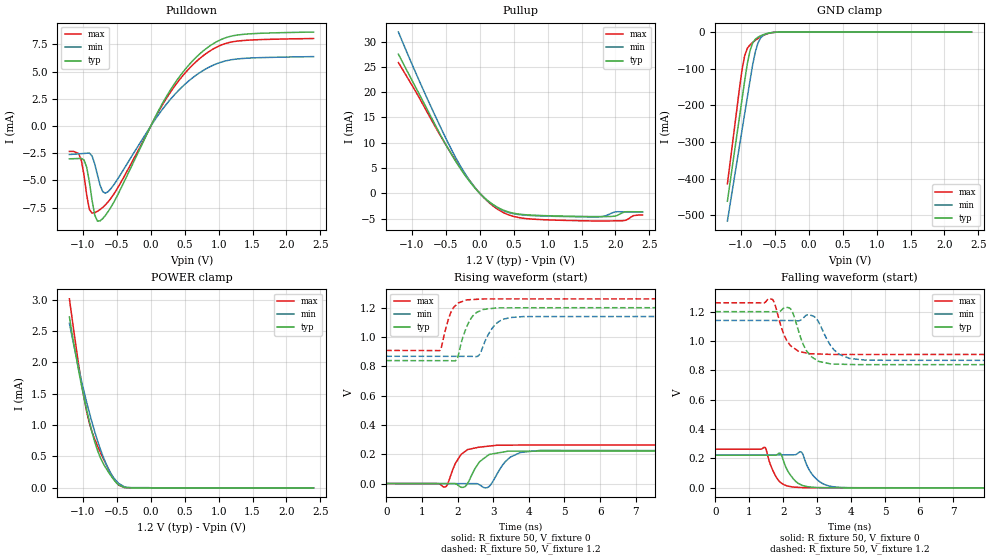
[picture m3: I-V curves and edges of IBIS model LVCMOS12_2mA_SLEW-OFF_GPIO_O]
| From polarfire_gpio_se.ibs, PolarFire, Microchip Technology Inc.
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|   Model LVCMOS12_2mA_SLEW-OFF_GPIO_O
[Model]   LVCMOS12_2mA_SLEW-OFF_GPIO_O
Model_type   Output
Polarity   Non-Inverting
Enable   Active-High
Vmeas =   0.6
Cref =   5p
Rref =   1M
|   typ   min   max
C_comp_pullup   2.605e-12   2.605e-12   2.76e-12
C_comp_pulldown  2.605e-12   2.605e-12   2.76e-12
[Temperature Range]  25C   100C   -40C
[Voltage Range]  1.2   1.14   1.26
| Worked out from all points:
|   slope of the pulldown table from 0 to 0.18 V, typ, clamps not added: 83 ohm
|   slope of the pullup table from 0 to 0.18 V, typ, clamps not added: 86.5 ohm
|   GND clamp passes 1 mA (typ) near -0.52 V on its own axis
|   POWER clamp passes 1 mA (typ) near -0.89 V on its own axis
|   rising waveform, R_fixture 50, V_fixture 0: 20-80 % time 401ps typ, 415ps min, 360ps max; typ from 0 V to 0.222 V
|   rising waveform, R_fixture 50, V_fixture 1.2: 20-80 % time 324ps typ, 370ps min, 269ps max; typ from 0.839 V to 1.2 V
|   falling waveform, R_fixture 50, V_fixture 0: 20-80 % time 351ps typ, 402ps min, 303ps max; typ from 0.222 V to 0 V
|   falling waveform, R_fixture 50, V_fixture 1.2: 20-80 % time 385ps typ, 449ps min, 353ps max; typ from 1.2 V to 0.839 V
[GND Clamp]
| Voltage   I(typ)   I(min)   I(max)
-1.2V     -461.6mA   -515.5mA   -414.1mA
-1.024V   -233.9mA   -313mA     -156.3mA
-984.4mV  -183.1mA   -267.7mA   -102.9mA
-945mV    -132.4mA   -222.5mA   -64.19mA
-905.6mV  -85.65mA   -177.3mA   -44.28mA
-866.2mV  -50.48mA   -132.2mA   -34.88mA
-826.9mV  -29.63mA   -88.81mA   -28.27mA
-787.5mV  -19.44mA   -53.53mA   -22.49mA
-748.1mV  -13.93mA   -29.25mA   -17.33mA
-669.4mV  -7.138mA   -8.749mA   -8.991mA
-433.1mV  -123uA     -169.9uA   -145.4uA
2.4V      0A         0A         0A
[POWER Clamp]
| Voltage   I(typ)   I(min)   I(max)
-1.2V     2.722mA    2.621mA    3.012mA
-1.142V   2.337mA    2.308mA    2.555mA
-1.024V   1.644mA    1.716mA    1.685mA
-945mV    1.238mA    1.362mA    1.214mA
-905.6mV  1.055mA    1.197mA    1.032mA
-826.9mV  734.5uA    894.9uA    775uA
-748.1mV  493.1uA    630.3uA    576.4uA
-590.6mV  198.3uA    234.5uA    226.1uA
-472.5mV  46.9uA     69.92uA    43.42uA
-393.7mV  7.199uA    19.02uA    5.897uA
-275.6mV  135nA      3.464uA    713.5nA
2.4V      0A         0A         0A
[Pullup]
| Voltage   I(typ)   I(min)   I(max)
-1.2V     27.53mA    31.91mA    25.87mA
-787.5mV  16.92mA    19.12mA    16.33mA
-354.4mV  6.31mA     7.042mA    6.437mA
-78.75mV  1.158mA    1.239mA    1.262mA
187.5mV   -2.153mA   -2.238mA   -2.418mA
450mV     -3.789mA   -3.896mA   -4.382mA
787.5mV   -4.337mA   -4.423mA   -5.119mA
1.751V    -4.613mA   -4.661mA   -5.485mA
1.988V    -4.533mA   -3.71mA    -5.455mA
2.106V    -3.839mA   -3.653mA   -5.428mA
2.263V    -3.652mA   -3.67mA    -4.429mA
2.4V      -3.666mA   -3.684mA   -4.306mA
[Pulldown]
| Voltage   I(typ)   I(min)   I(max)
-1.2V     -3.01mA    -2.609mA   -2.328mA
-1.063V   -2.981mA   -2.553mA   -2.523mA
-984.4mV  -3.121mA   -2.516mA   -4.527mA
-905.6mV  -5.132mA   -2.483mA   -7.666mA
-826.9mV  -8.174mA   -3.482mA   -7.96mA
-748.1mV  -8.716mA   -5.422mA   -7.67mA
-669.4mV  -8.208mA   -6.166mA   -7.241mA
-590.6mV  -7.483mA   -5.768mA   -6.66mA
225mV     2.654mA    1.965mA    2.495mA
750mV     6.782mA    5.02mA     6.35mA
1.239V    8.326mA    6.139mA    7.775mA
2.4V      8.637mA    6.378mA    8.041mA
[Ramp]
dV/dt_r   0.13305/0.400691n  0.134808/0.414574n  0.157753/0.360389n
dV/dt_f   0.216628/0.384966n  0.163062/0.448816n  0.2111/0.352531n
R_load = 50
[Rising Waveform]
R_fixture = 50
V_fixture = 0
V_fixture_min = 0
V_fixture_max = 0
| Time   V(typ)   V(min)   V(max)
0s        21.82nV    34.2nV     29.76nV
1.663ns   -768.5uV   -579.9uV   -22.85mV
1.942ns   -1.74mV    -677.1uV   138.7mV
2.165ns   -26.03mV   -754.9uV   210.1mV
2.618ns   148.6mV    -8.759mV   248.2mV
2.839ns   189.4mV    -27.5mV    254.1mV
3.106ns   207.4mV    63.56mV    261.3mV
3.478ns   220.8mV    179.8mV    261.9mV
4.342ns   220.9mV    226.4mV    262.7mV
10ns      221.8mV    224.7mV    262.9mV
[Rising Waveform]
R_fixture = 50
V_fixture = 1.2
V_fixture_min = 1.14
V_fixture_max = 1.26
| Time   V(typ)   V(min)   V(max)
0s        838.9mV    868.2mV    908.2mV
1.496ns   838.3mV    868mV      906.5mV
1.792ns   838.2mV    867.9mV    1.154V
1.979ns   846.7mV    867.9mV    1.224V
2.257ns   1.068V     867.8mV    1.253V
2.565ns   1.171V     868.4mV    1.257V
2.716ns   1.187V     936.4mV    1.259V
3.045ns   1.197V     1.081V     1.26V
3.478ns   1.199V     1.132V     1.26V
10ns      1.2V       1.14V      1.26V
[Falling Waveform]
R_fixture = 50
V_fixture = 0
V_fixture_min = 0
V_fixture_max = 0
| Time   V(typ)   V(min)   V(max)
0s        221.8mV    224.5mV    262.9mV
1.465ns   222.1mV    224.9mV    274.7mV
1.663ns   222.2mV    224.9mV    135.8mV
1.919ns   234.3mV    225mV      36.92mV
2.121ns   121.2mV    225mV      12.94mV
2.304ns   59.83mV    225.1mV    4.932mV
2.53ns    20.1mV     244mV      2.012mV
2.903ns   3.496mV    77.88mV    717.7uV
3.455ns   -57.26uV   8.063mV    661.9uV
10ns      -1.494uV   -7.865uV   -66.47nV
[Falling Waveform]
R_fixture = 50
V_fixture = 1.2
V_fixture_min = 1.14
V_fixture_max = 1.26
| Time   V(typ)   V(min)   V(max)
0s        1.2V       1.14V      1.26V
1.674ns   1.199V     1.139V     1.284V
2.176ns   1.225V     1.139V     980.7mV
2.281ns   1.194V     1.139V     957.2mV
2.606ns   968.2mV    1.16V      921.6mV
2.794ns   901mV      1.176V     913mV
2.99ns    868.2mV    1.149V     911.5mV
3.493ns   842.7mV    940.1mV    908.1mV
3.951ns   840.1mV    881.2mV    908.1mV
10ns      839mV      868.2mV    908.2mV
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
